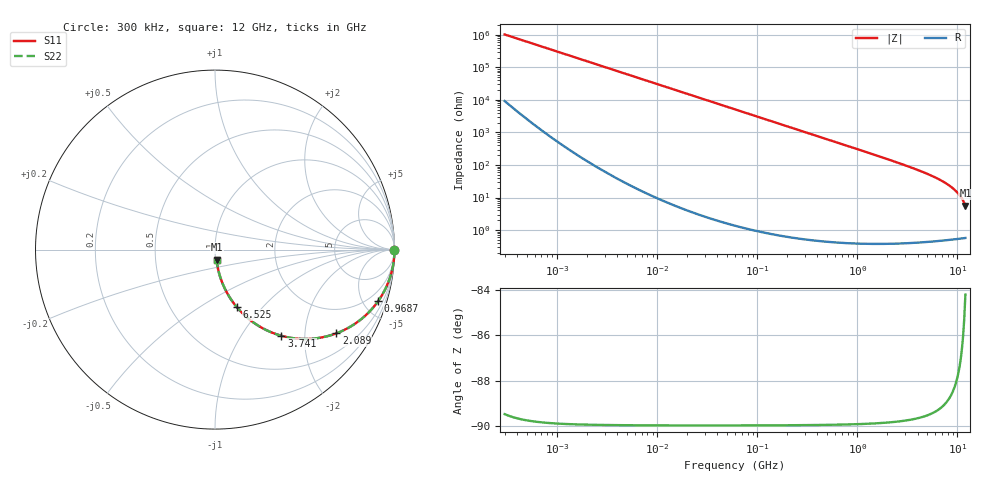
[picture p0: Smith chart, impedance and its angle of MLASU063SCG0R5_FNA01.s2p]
! MLASU063SCG0R5_FNA01  S-PARAMETER MODEL  ( Standard Model )
! Model Generated by TAIYO YUDEN Corporation (http://www.ty-top.com)
! Version 1.0
! TAIYO YUDEN Control No. 240819
! Copyright(c) 2024 TAIYO YUDEN CO.,LTD. All Rights Reserved.
! Product Description (link to TY-COMPAS)
! https://ds.yuden.co.jp/TYCOMPAS/or/detail?pn=MLASU063SCG0R5CFNA01&u=M
! Products Name : Multilayer Ceramic Capacitors
! Characteristics :
!  Capacitance : 0.5 [pF] , Rated Voltage : 50 [V] , TCC : CG / C0G
!  Case Size : 0.6 x 0.3 / 0.024 x 0.012 [mm/inch] , Thickness : 0.3 / 0.012 [mm/inch]
!  (Conditions: Temperature = 25 [degC] , DC Bias Voltage = 0 [V])
! External Node Assignments :
!  1  o---| |---o  2
! GND o---------o GND
! Frequency Range : 0.3MHz  -  12000MHz  [ 401 STEP ]
# MHZ S RI R 50
! Freq[MHz].  S11 Real  S11 Imag  S21 Real  S21 Imag  S12 Real  S12 Imag  S22 Real  S22 Imag
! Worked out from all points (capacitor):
!   401 points, 300 kHz to 12 GHz, reference 50 ohm
!   read as one part in series: C = 514 fF near 316.3 kHz
!   lowest |Z| = 5.64 ohm at 12 GHz (marker M1)
!   S11 on the Smith chart (normalised r, x): 300 kHz: open; 968.7 MHz: 1.01, -6.36; 2.089 GHz: 1.01, -2.90; 3.741 GHz: 1.01, -1.53; 6.525 GHz: 1.01, -0.73; 12 GHz: 1.01, -0.11
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0.3  1 -9.68e-05  8.81e-07 9.68e-05  8.81e-07 9.68e-05  1 -9.68e-05
0.333535  1 -0.000108  8.31e-07 0.000108  8.31e-07 0.000108  1 -0.000108
1.769972  1 -0.000571  8.67e-07 0.000571  8.67e-07 0.000571  1 -0.000571
10.44266  1 -0.00337  1.24e-05 0.00337  1.24e-05 0.00337  1 -0.00337
60  0.9996 -0.0194  0.00038 0.0194  0.00038 0.0194  0.9996 -0.0194
164.1901  0.9972 -0.0529  0.00282 0.0529  0.00282 0.0529  0.9972 -0.0529
353.9943  0.987 -0.1129  0.013 0.1129  0.013 0.1129  0.987 -0.1129
634.0297  0.9595 -0.1968  0.0405 0.1968  0.0405 0.1968  0.9595 -0.1968
968.706  0.9098 -0.2858  0.0902 0.2858  0.0902 0.2858  0.9098 -0.2858
1441.349  0.8183 -0.3847  0.1817 0.3847  0.1817 0.3847  0.8183 -0.3847
1735.023  0.7547 -0.4292  0.2453 0.4292  0.2453 0.4292  0.7547 -0.4292
2088.533  0.6767 -0.4664  0.3233 0.4664  0.3233 0.4664  0.6767 -0.4664
2795.104  0.5296 -0.4973  0.4704 0.4973  0.4704 0.4973  0.5296 -0.4973
3740.715  0.37 -0.4801  0.63 0.4801  0.63 0.4801  0.37 -0.4801
5006.236  0.2241 -0.413  0.7759 0.413  0.7759 0.413  0.2241 -0.413
6524.734  0.1206 -0.3194  0.8794 0.3194  0.8794 0.3194  0.1206 -0.3194
8064.993  0.0622 -0.2317  0.9378 0.2317  0.9378 0.2317  0.0622 -0.2317
8732.115  0.0458 -0.1972  0.9542 0.1972  0.9542 0.1972  0.0458 -0.1972
9454.42  0.0324 -0.1622  0.9676 0.1622  0.9676 0.1622  0.0324 -0.1622
10511.28  0.0188 -0.1149  0.9812 0.1149  0.9812 0.1149  0.0188 -0.1149
11686.27  0.0102 -0.0672  0.9898 0.0672  0.9898 0.0672  0.0102 -0.0672
12000  0.00876 -0.0553  0.9912 0.0553  0.9912 0.0553  0.00876 -0.0553
